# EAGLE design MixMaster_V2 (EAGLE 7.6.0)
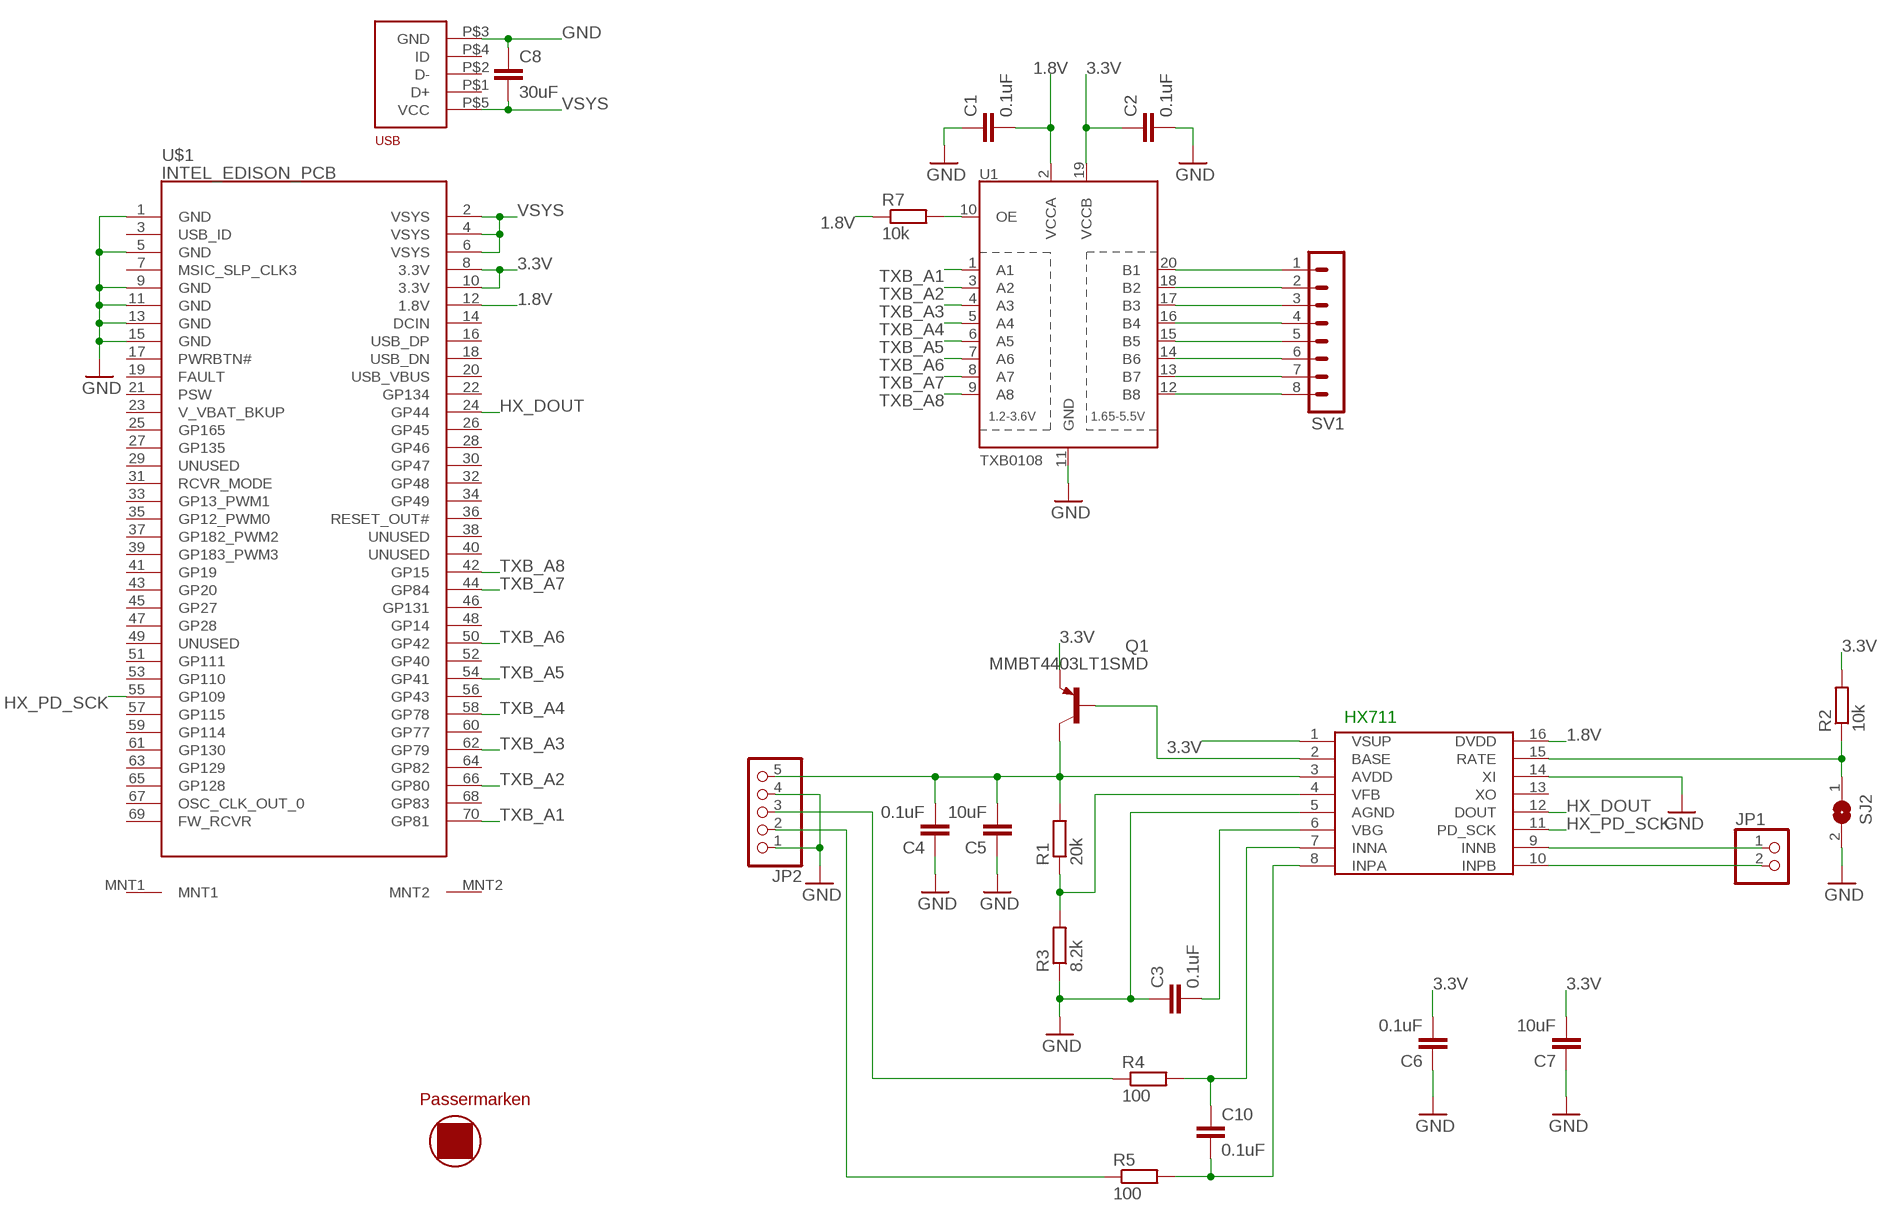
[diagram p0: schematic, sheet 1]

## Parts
C1  0.1uF  C-EUC0805  [C0805]
C2  0.1uF  C-EUC0805  [C0805]
C3  0.1uF  C-EUC0805  [C0805]
C4  0.1uF  C-EUC0805  [C0805]
C5  10uF  C-EUC0805  [C0805]
C6  0.1uF  C-EUC0805  [C0805]
C7  10uF  C-EUC0805  [C0805]
C8  30uF  C-EUC0805  [C0805]
C10  0.1uF  C-EUC0805  [C0805]
JP1  PINHD-1X2  [1X02]
JP2  PINHD-1X5  [1X05]
Q1  MMBT4403LT1SMD  [SOT23-BEC]
R1  20k  R-EU_R0805  [R0805]
R2  10k  R-EU_R0805  [R0805]
R3  8.2k  R-EU_R0805  [R0805]
R4  100  R-EU_R0805  [R0805]
R5  100  R-EU_R0805  [R0805]
R7  10k  R-EU_R0805  [R0805]
SJ2  SJ  [SJ]
SV1  MA08-1  [MA08-1]
U1  TXB0108  [TSSOP20]
U$1  INTEL_EDISON_PCB  [INTEL_EDISON]
U$2  HX711  [SO16]
U$3  USB  [USB]
U$4  PASSERMARKEN  [MASTERSUBSTRAT-MITPASSERMARKEN]

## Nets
1.8V: C1.2 R7.1 U1.2(VCCA) U$1.12(1.8V) U$2.16(DVDD)
3.3V: C2.1 C6.2 C7.2 Q1.E R2.2 U1.19(VCCB) U$1.8(3.3V) U$1.10(3.3V) U$2.1(VSUP)
GND: C1.1 C2.2 C3.1 C4.1 C5.1 C6.1 C7.1 C8.1 JP2.1 JP2.4 R3.1 SJ2.2 U1.11(GND) U$1.1(GND) U$1.5(GND) U$1.9(GND) U$1.11(GND) U$1.13(GND) U$1.15(GND) U$2.5(AGND) U$2.14(XI) U$3.P$3(GND)
HX_DOUT: U$1.24(GP44) U$2.12(DOUT)
HX_PD_SCK: U$1.55(GP109) U$2.11(PD_SCK)
N$1: R7.2 U1.10(OE)
N$2: SV1.1 U1.20(B1)
N$3: SV1.2 U1.18(B2)
N$4: SV1.3 U1.17(B3)
N$5: SV1.4 U1.16(B4)
N$6: SV1.5 U1.15(B5)
N$7: SV1.6 U1.14(B6)
N$8: SV1.7 U1.13(B7)
N$9: SV1.8 U1.12(B8)
N$11: Q1.B U$2.2(BASE)
N$12: R2.1 SJ2.1 U$2.15(RATE)
N$13: JP1.1 U$2.9(INNB)
N$14: JP1.2 U$2.10(INPB)
N$15: R1.1 R3.2 U$2.4(VFB)
N$16: JP2.2 R5.1
N$17: C3.2 U$2.6(VBG)
N$18: C10.1 R4.2 U$2.7(INNA)
N$19: C10.2 R5.2 U$2.8(INPA)
N$20: JP2.3 R4.1
N$21: C4.2 C5.2 JP2.5 Q1.C R1.2 U$2.3(AVDD)
TXB_A1: U1.1(A1) U$1.70(GP81)
TXB_A2: U1.3(A2) U$1.66(GP80)
TXB_A3: U1.4(A3) U$1.62(GP79)
TXB_A4: U1.5(A4) U$1.58(GP78)
TXB_A5: U1.6(A5) U$1.54(GP41)
TXB_A6: U1.7(A6) U$1.50(GP42)
TXB_A7: U1.8(A7) U$1.44(GP84)
TXB_A8: U1.9(A8) U$1.42(GP15)
VSYS: C8.2 U$1.2(VSYS) U$1.4(VSYS) U$1.6(VSYS) U$3.P$5(VCC)
Unconnected: U$1.3(USB_ID) U$1.7(MSIC_SLP_CLK3) U$1.14(DCIN) U$1.16(USB_DP) U$1.17(PWRBTN#) U$1.18(USB_DN) U$1.19(FAULT) U$1.20(USB_VBUS) U$1.21(PSW) U$1.22(GP134) U$1.23(V_VBAT_BKUP) U$1.25(GP165) U$1.26(GP45) U$1.27(GP135) U$1.28(GP46) U$1.29(UNUSED) U$1.30(GP47) U$1.31(RCVR_MODE) U$1.32(GP48) U$1.33(GP13_PWM1) U$1.34(GP49) U$1.35(GP12_PWM0) U$1.36(RESET_OUT#) U$1.37(GP182_PWM2) U$1.38(UNUSED) U$1.39(GP183_PWM3) U$1.40(UNUSED) U$1.41(GP19) U$1.43(GP20) U$1.45(GP27) U$1.46(GP131) U$1.47(GP28) U$1.48(GP14) U$1.49(UNUSED) U$1.51(GP111) U$1.52(GP40) U$1.53(GP110) U$1.56(GP43) U$1.57(GP115) U$1.59(GP114) U$1.60(GP77) U$1.61(GP130) U$1.63(GP129) U$1.64(GP82) U$1.65(GP128) U$1.67(OSC_CLK_OUT_0) U$1.68(GP83) U$1.69(FW_RCVR) U$1.MNT1 U$1.MNT2 U$2.13(XO) U$3.P$1(D+) U$3.P$2(D-) U$3.P$4(ID)

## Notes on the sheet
- HX711

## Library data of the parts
C1-C8 C10 = rcl:C-EU: CAPACITOR, European symbol
JP1 = pinhead:PINHD-1X2: PIN HEADER
JP2 = pinhead:PINHD-1X5: PIN HEADER
Q1 = transistor-pnp:MMBT4403*: PNP Transistror
R1-R5 R7 = rcl:R-EU_: RESISTOR, European symbol
SJ2 = jumper:SJ: SMD solder JUMPER
SV1 = con-lstb:MA08-1: PIN HEADER; OC_FARNELL: unknown; OC_NEWARK: unknown
U1 = TXB0108:TXB0108: 8-Bit Bi-Directional Level Shifter 1.2V-3.6V (VCCA) to 1.65V-5.5V (VCCB) bi-directional level shifter with auto direction sensing. Max data rate - VCCA 1.8V: 20Mbps (50ns), VCCA 3.3V: 100Mbps (10ns) Digikey: 296-21527-1-ND; AVAILABILITY: Unavailable; DESCRIPTION: 8-Bit Bidirectional Voltage-Level Translator with Auto Direction Sensing and +/-15-kV ESD Protect; MF: Texas Instruments; MP: TXB0108; PACKAGE: None; PRICE: None
U$1 = e14_Intel_Edison_RevA:INTEL_EDISON_PCB: Intel Edison Compute Module. Ideal for creating your own PCB to host an Edison. Created for www.element14.com by Dave of Young Circuit Designs. Note: 70-pin connector on the Edison is a 1.5mm-tall Hirose plug DF40C-70DP-0.4V(51) Mating Hirose receptacle connectors of varying heights include the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
U$2 = HX711:HX711
U$3 = USB_Buchse:USB
U$4 = lmhs:PASSERMARKEN

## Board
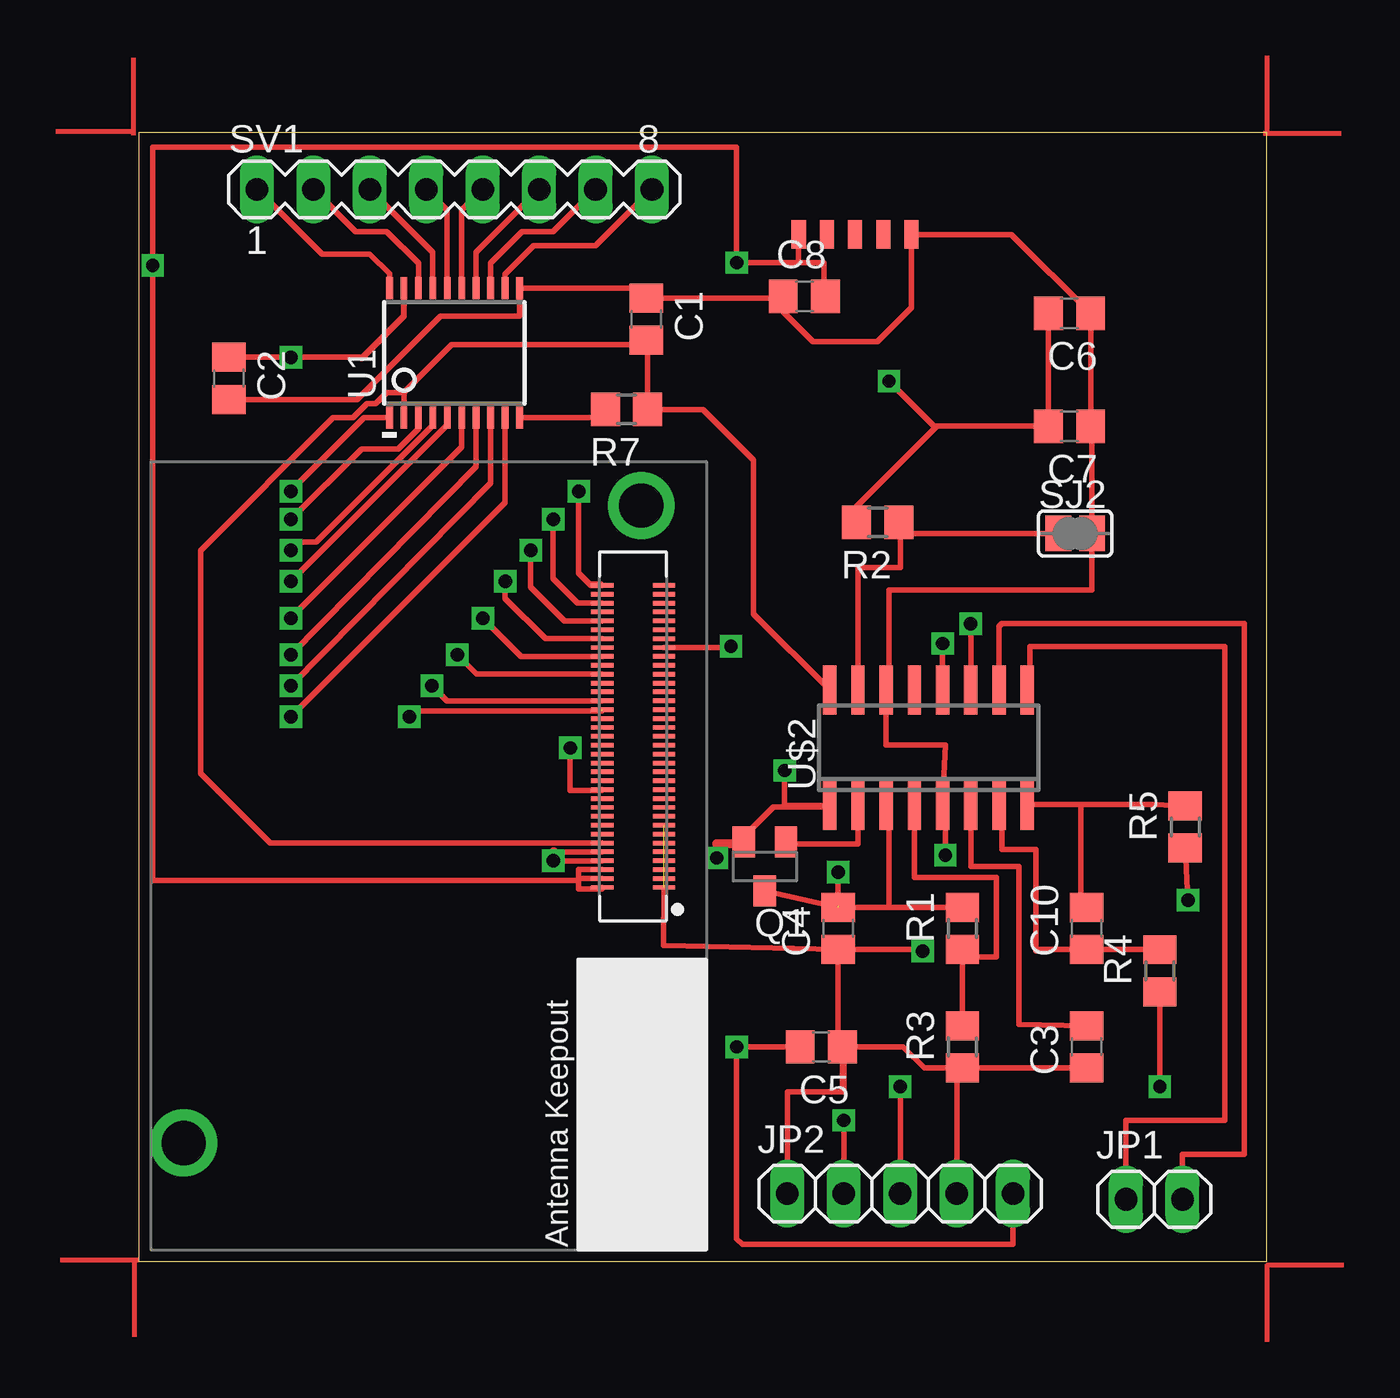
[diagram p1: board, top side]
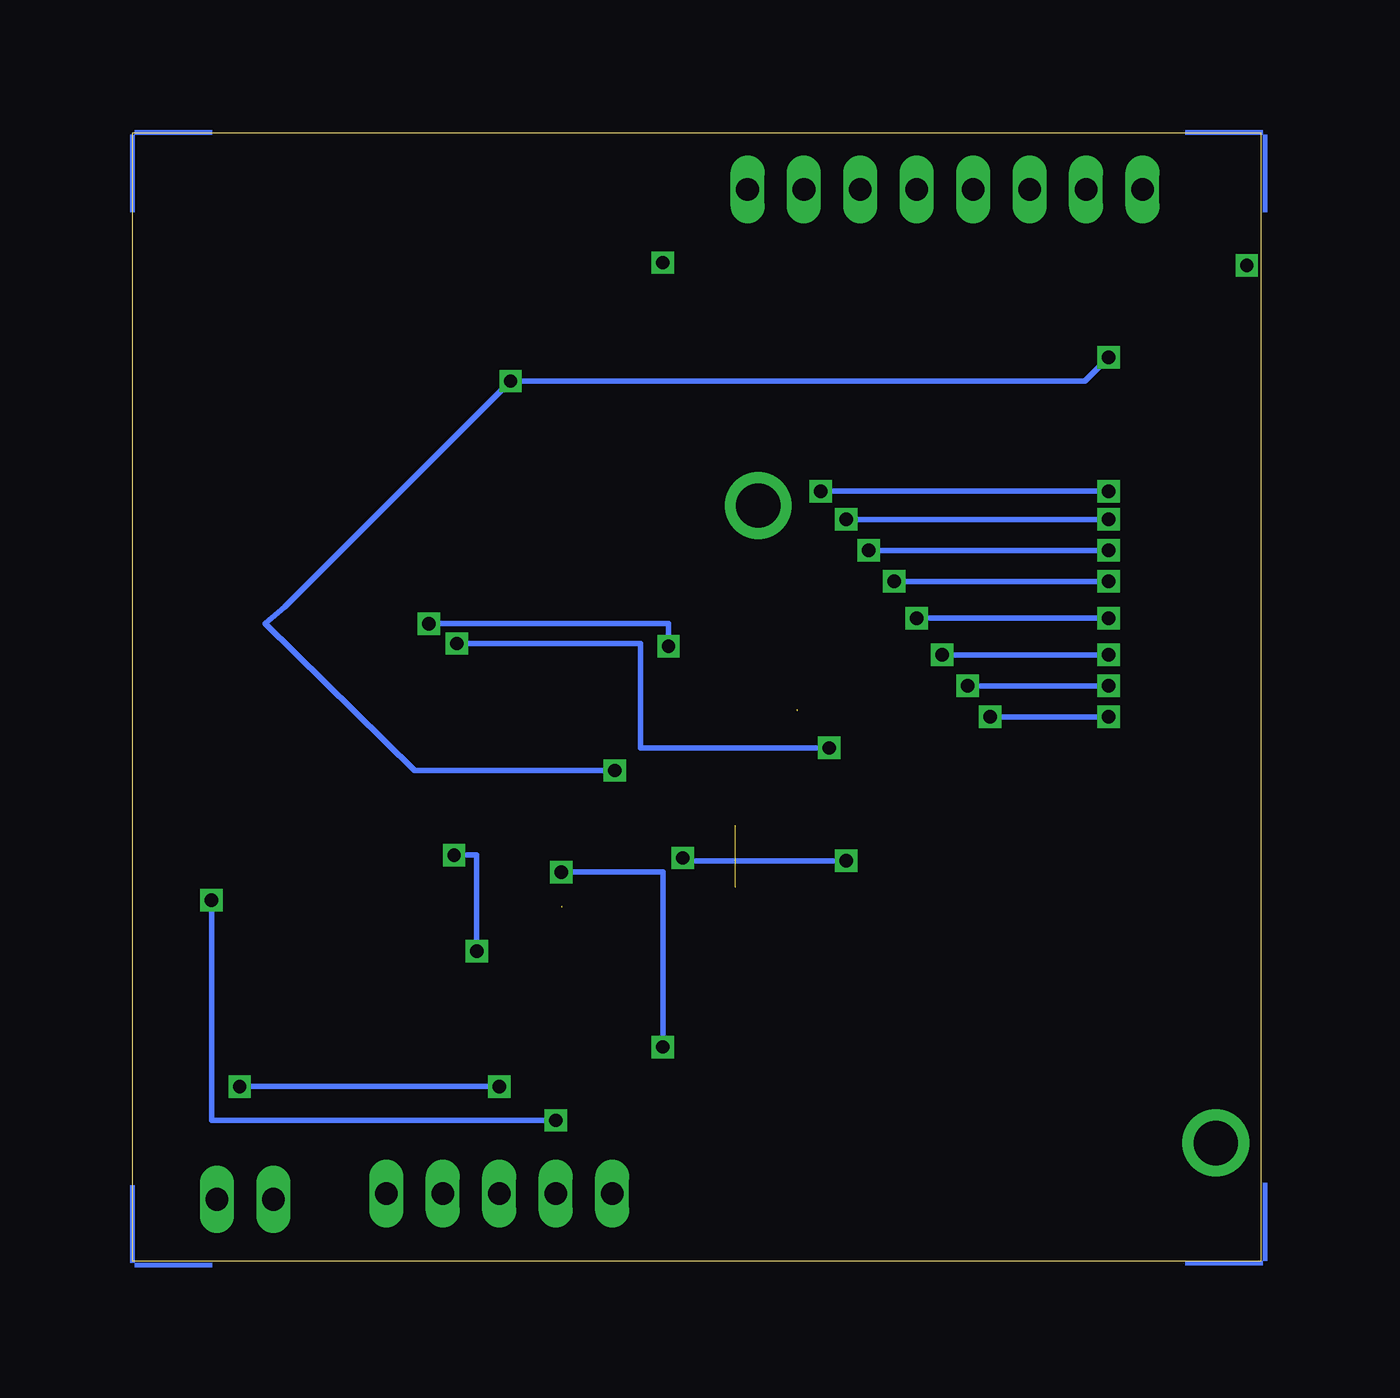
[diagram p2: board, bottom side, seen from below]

Size 50.8 x 50.8 mm. Coordinates in mm from the lower left corner, seen from the top.
Outline: 0,0 50.8,0 50.8,50.8 0,50.8 0,0
Copper layers (1*16): Top 0.035mm / dielectric 1.5mm / Bottom 0.035mm
Design rules "default": minimum track width 10mil, minimum drill 24mil, track to track 8mil, track to pad 8mil, pad to pad 8mil, via to via 8mil, smd to smd 8mil, copper to edge 40mil, drill to drill 8mil, minimum pad ring 10mil, minimum via ring 8mil, stop-mask expansion 4mil, vias tented up to drill 0mil, thermal gap 10mil

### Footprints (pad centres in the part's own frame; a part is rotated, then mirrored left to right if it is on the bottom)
C0805 = smd 1.3 x 1.5: 1 -0.95,0; 2 0.95,0
1X02 = drill 1.016 long: 1 -1.27,0; 2 1.27,0
1X05 = drill 1.016 long: 1 -5.08,0; 2 -2.54,0; 3 0,0; 4 2.54,0; 5 5.08,0
SOT23-BEC = smd 1 x 1.4: B -0.95,-1.1; C 0,1.1; E 0.95,-1.1
R0805 = smd 1.3 x 1.5: 1 -0.95,0; 2 0.95,0
SJ = smd 1.168 x 1.6: 1 -0.762,0; 2 0.762,0
MA08-1 = drill 1.016 long: 1 -8.89,0; 2 -6.35,0; 3 -3.81,0; 4 -1.27,0; 5 1.27,0; 6 3.81,0; 7 6.35,0; 8 8.89,0
TSSOP20 = smd 0.305 x 0.991: 1 -2.925,-2.918; 2 -2.275,-2.918; 3 -1.625,-2.918; 4 -0.975,-2.918; 5 -0.325,-2.918; 6 0.325,-2.918; 7 0.975,-2.918; 8 1.625,-2.918; 9 2.275,-2.918; 10 2.925,-2.918; 11 2.925,2.918; 12 2.275,2.918; 13 1.625,2.918; 14 0.975,2.918; 15 0.325,2.918; 16 -0.325,2.918; 17 -0.975,2.918; 18 -1.625,2.918; 19 -2.275,2.918; 20 -2.925,2.918
INTEL_EDISON = smd 1 x 0.2: 1 21.62,11.5; 2 18.84,11.5; 3 21.62,11.9; 4 18.84,11.9; 5 21.62,12.3; 6 18.84,12.3; 7 21.62,12.7; 8 18.84,12.7; 9 21.62,13.1; 10 18.84,13.1; 11 21.62,13.5; 12 18.84,13.5; 13 21.62,13.9; 14 18.84,13.9; 15 21.62,14.3; 16 18.84,14.3; 17 21.62,14.7; 18 18.84,14.7; 19 21.62,15.1; 20 18.84,15.1; 21 21.62,15.5; 22 18.84,15.5; 23 21.62,15.9; 24 18.84,15.9; 25 21.62,16.3; 26 18.84,16.3; 27 21.62,16.7; 28 18.84,16.7; 29 21.62,17.1; 30 18.84,17.1; 31 21.62,17.5; 32 18.84,17.5; 33 21.62,17.9; 34 18.84,17.9; 35 21.62,18.3; 36 18.84,18.3; 37 21.62,18.7; 38 18.84,18.7; 39 21.62,19.1; 40 18.84,19.1; 41 21.62,19.5; 42 18.84,19.5; 43 21.62,19.9; 44 18.84,19.9; 45 21.62,20.3; 46 18.84,20.3; 47 21.62,20.7; 48 18.84,20.7; 49 21.62,21.1; 50 18.84,21.1; 51 21.62,21.5; 52 18.84,21.5; 53 21.62,21.9; 54 18.84,21.9; 55 21.62,22.3; 56 18.84,22.3; 57 21.62,22.7; 58 18.84,22.7; 59 21.62,23.1; 60 18.84,23.1; 61 21.62,23.5; 62 18.84,23.5; 63 21.62,23.9; 64 18.84,23.9; 65 21.62,24.3; 66 18.84,24.3; 67 21.62,24.7; 68 18.84,24.7; 69 21.62,25.1; 70 18.84,25.1 | drill 2: MNT1 0,0; MNT2 20.6,28.69
SO16 = smd 0.6 x 2.2: 1 -4.445,-2.6; 2 -3.175,-2.6; 3 -1.905,-2.6; 4 -0.635,-2.6; 5 0.635,-2.6; 6 1.905,-2.6; 7 3.175,-2.6; 8 4.445,-2.6; 9 4.445,2.6; 10 3.175,2.6; 11 1.905,2.6; 12 0.635,2.6; 13 -0.635,2.6; 14 -1.905,2.6; 15 -3.175,2.6; 16 -4.445,2.6
USB = smd 1.27 x 0.635: P$1 3.81,0; P$2 3.81,1.27; P$3 3.81,2.54; P$4 3.81,-1.27; P$5 3.81,-2.54

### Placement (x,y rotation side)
C1  22.86,42.42 270 top
C2  4.06,39.75 270 top
C3  42.67,9.65 90 top
C4  31.5,14.99 90 top
C5  30.73,9.65 180 top
C6  41.91,42.67 180 top
C7  41.91,37.59 180 top
C8  29.97,43.43 0 top
C10  42.67,14.99 90 top
JP1  45.72,2.79 0 top
JP2  34.29,3.05 0 top
Q1  28.19,17.78 180 top
R1  37.08,14.99 90 top
R2  33.27,33.27 180 top
R3  37.08,9.65 90 top
R4  45.97,13.08 90 top
R5  47.12,19.56 90 top
R7  21.97,38.35 180 top
SJ2  42.16,32.77 0 top
SV1  14.22,48.26 0 top
U1  14.22,40.89 0 top
U$1  2.03,5.33 0 top
U$2  35.56,23.11 0 top
U$3  32.26,50.04 270 top
U$4  not placed on the board

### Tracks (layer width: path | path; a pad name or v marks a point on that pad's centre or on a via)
1.8V
  Top 0.254: U1.2 11.95,39.13 | 11.95,39.13 14.1,41.27 22.67,41.27 C1.2 22.92,41.41 R7.1 25.4,38.35 27.69,36.07 27.69,29.14 U$2.16 | U$1.12 5.93,18.83 2.79,21.97 2.79,32 8.76,37.97 9.65,37.97 10.29,38.61 10.67,38.61 11.18,39.12 11.94,39.12 11.95,39.13
3.3V  (via drill 0.6)
  Top 0.254: C6.2 C7.2 35.94,37.59 | 18.69,18.43 U$1.10 | U$1.8 v18.67,18.03 | 10.03,40.64 11.95,42.56 U1.19 11.94,43.8 11.94,42.55 10.09,40.7 v6.86,40.7 C2.1 | 35.94,37.59 32.32,33.98 R2.2 32.26,33.27 | 35.94,37.59 35.81,37.59 v33.78,39.62 | Q1.E 27.24,19.12 28.57,20.45 29.08,20.45 | 29.08,20.45 31.05,20.45 U$2.1 29.15,20.51 29.08,20.45 | 29.08,20.45 v29.08,22.1
  Top 0.406: Q1.E 27.16,18.8 26.04,18.8 v26.04,18.16 | v18.67,18.03 18.67,18.41 18.69,18.43
  Bottom 0.254: 25.91,18.03 v18.67,18.03 | v6.86,40.7 7.93,39.62 v33.78,39.62 43.94,29.46 44.83,28.7 38.1,22.1 v29.08,22.1
  Bottom 0.406: v26.04,18.16 25.91,18.03
GND  (via drill 0.6)  (5 unrouted)
  Top 0.254: SJ2.2 42.93,37.59 C7.1 C6.1 39.3,46.23 U$3.P$3 34.8,42.93 33.27,41.4 30.35,41.4 29.02,42.73 C8.1 28.96,43.37 C1.1 22.42,43.81 U1.11 17.14,42.55 13.59,42.55 9.85,38.8 C2.2 | SJ2.2 43.18,32.77 | SJ2.2 42.93,30.23 33.78,30.23 33.78,25.71 U$2.14 33.66,23.24 36.32,23.24 U$2.5 36.32,20.39 v36.32,18.29 | JP2.4 36.83,8.45 R3.1 | R3.1 C3.1 | U$1.1 23.62,14.22 C4.1 | v35.31,13.97 35.24,14.04 C4.1 | C4.1 31.5,9.84 C5.1 31.68,7.69 31.75,7.62 | JP2.1 29.21,7.62 31.75,7.62 | 31.75,7.62 31.75,9.65 34.42,9.65 35.37,8.7 R3.1
  Bottom 0.254: v36.32,18.29 35.31,18.29 v35.31,13.97
HX_DOUT  (via drill 0.6)
  Top 0.254: U$2.12 v36.2,27.81 | v19.43,23.11 19.43,21.21 20.87,21.21 U$1.24
  Bottom 0.254: v36.2,27.81 27.94,27.81 27.94,23.11 v19.43,23.11
HX_PD_SCK  (via drill 0.6)
  Top 0.254: U$1.55 26.67,27.63 v26.67,27.69 | v37.47,28.7 U$2.11
  Bottom 0.254: v26.67,27.69 26.67,28.7 v37.47,28.7
N$1
  Top 0.254: U1.10 20.64,37.98 R7.2
N$2
  Top 0.254: U1.20 11.3,44.45 10.41,45.34 8.26,45.34 SV1.1
N$3
  Top 0.254: U1.18 12.6,44.93 11.18,46.35 9.78,46.35 SV1.2
N$4
  Top 0.254: U1.17 13.25,45.42 SV1.3
N$5
  Top 0.254: U1.16 13.9,47.31 SV1.4
N$6
  Top 0.254: U1.15 14.55,47.31 SV1.5
N$7
  Top 0.254: U1.14 15.2,45.42 SV1.6
N$8
  Top 0.254: U1.13 15.85,44.93 17.27,46.35 18.67,46.35 SV1.7
N$9
  Top 0.254: U1.12 16.5,44.44 17.78,45.72 20.57,45.72 SV1.8
N$10
  Top 0.254: 20.83,30.48 20.32,30.48 19.81,30.99 19.81,34.67
N$11
  Top 0.254: Q1.B 28.97,18.8 32.38,18.8 U$2.2
N$12
  Top 0.254: SJ2.1 34.22,32.77 R2.1 34.29,33.27 34.29,31.24 32.38,31.24 U$2.15
N$13
  Top 0.254: U$2.9 40.13,25.84 40.13,27.69 48.9,27.69 48.9,6.35 44.45,6.35 JP1.1
N$14
  Top 0.254: JP1.2 46.99,4.83 49.78,4.83 49.78,28.7 38.86,28.7 38.73,28.57 U$2.10
N$15
  Top 0.254: R3.2 37.08,13.72 | 37.08,13.72 R1.1 | U$2.4 34.92,17.27 38.61,17.27 38.61,13.72 37.08,13.72
N$16  (via drill 0.6)
  Top 0.254: JP2.2 v31.75,6.35 | v47.24,16.26 R5.1
  Bottom 0.254: v31.75,6.35 47.24,6.35 v47.24,16.26
N$17
  Top 0.254: U$2.6 37.47,17.78 39.62,17.78 39.62,10.67 C3.2
N$18
  Top 0.254: U$2.7 38.86,20.39 38.86,18.54 40.39,18.54 40.39,13.97 40.45,14.04 C10.1 45.59,14.04 R4.2
N$19
  Top 0.254: U$2.8 40.06,20.57 42.42,20.57 | 42.42,20.57 45.65,20.57 R5.2 | C10.2 42.42,16.19 42.42,20.57
N$20  (via drill 0.6)
  Top 0.254: R4.1 v45.97,7.87 | v34.29,7.87 JP2.3
  Bottom 0.254: v45.97,7.87 v34.29,7.87
N$21  (via drill 0.6)  (1 unrouted)
  Top 0.254: 31.5,16 v31.5,17.53 | Q1.C C4.2 33.78,15.94 | 33.78,15.94 R1.2 | U$2.3 33.78,20.39 33.78,15.94 | C5.2 v26.92,9.65 26.92,1.02 27.18,0.76 39.37,0.76 JP2.5
  Bottom 0.254: v31.5,17.53 26.92,17.53 v26.92,9.65
TXB_A1  (via drill 0.6)
  Top 0.254: U$1.70 20.37,30.43 19.81,30.99 v19.81,34.67 | U1.1 10.16,37.98 v6.86,34.67
  Bottom 0.254: v6.86,34.67 v19.81,34.67
TXB_A2  (via drill 0.6)
  Top 0.254: U$1.66 19.77,29.63 18.67,30.73 v18.67,33.4 | U1.3 12.6,37.49 11.68,36.58 10.03,36.58 v6.86,33.4
  Bottom 0.254: v18.67,33.4 18.03,33.4 17.91,33.4 v6.86,33.4
TXB_A3  (via drill 0.6)
  Top 0.254: U$1.62 19.17,28.83 17.65,30.35 v17.65,32 | U1.4 13.25,37.63 8,32.38 7.24,32.38 v6.86,32
  Bottom 0.254: v17.65,32 17.14,32 17.02,32 v6.86,32
TXB_A4  (via drill 0.6)
  Top 0.254: U$1.58 18.32,28.03 16.51,29.84 v16.51,30.61 | U1.5 13.9,37.65 v6.86,30.61
  Bottom 0.254: v6.86,30.61 v16.51,30.61
TXB_A5  (via drill 0.6)
  Top 0.254: U$1.54 17.22,27.23 v15.49,28.96 | U1.6 14.55,36.65 v6.86,28.96
  Bottom 0.254: v15.49,28.96 14.99,28.96 14.86,28.96 v6.86,28.96
TXB_A6  (via drill 0.6)
  Top 0.254: U$1.50 15.22,26.43 v14.35,27.3 | U1.7 15.2,35.77 v6.86,27.3
  Bottom 0.254: v6.86,27.3 v14.35,27.3
TXB_A7  (via drill 0.6)
  Top 0.254: U$1.44 13.88,25.23 v13.21,25.91 | U1.8 15.85,35.03 v6.86,25.91
  Bottom 0.254: v6.86,25.91 v13.21,25.91
TXB_A8  (via drill 0.6)  (1 unrouted)
  Top 0.254: 20.87,24.77 12.45,24.77 v12.19,24.51 | U1.9 16.5,34.15 v6.86,24.51
  Bottom 0.254: v6.86,24.51 v12.19,24.51
VSYS  (via drill 0.6)
  Top 0.254: U$1.6 19.81,17.63 19.81,17.23 | 19.81,17.23 19.81,17.14 | 19.81,17.14 19.81,16.76 20.87,16.76 U$1.2 | U$1.4 19.81,17.23 | 29.72,44.96 30.86,44.96 30.86,43.43 C8.2 | 29.72,44.96 U$3.P$5 | 29.72,44.96 v26.92,44.96 26.92,50.16 0.64,50.16 v0.64,44.83 0.64,17.14 16.76,17.14 19.81,17.14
